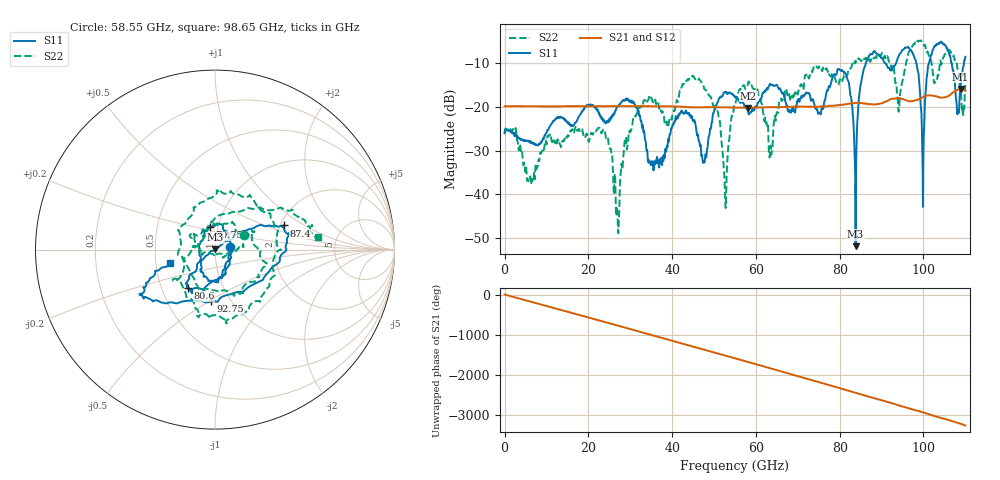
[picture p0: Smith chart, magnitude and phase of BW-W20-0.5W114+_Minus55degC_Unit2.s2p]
!Mini-Circuits Laboratory
!S-Parameters
!Model: BW-W20-0.5W114+
!Run / Lot / Date Code: QN2409253 /  / N/A
!Fixture:
!Network Analyzer: PNA-X N5242B - 423 4 ports (COM/DCOM);  Serial number: 74408
!Date: 3/8/2024 at 1:33:00 PM
!No.: Unit# 4 (U2  -55C)
!Tested with:
# Hz  S  dB  R  50
!Frequency  S11 dB  S11 Deg  S21 dB  S21 Deg  S12 dB  S12 Deg  S22 dB  S22 Deg
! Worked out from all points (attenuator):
!   2208 points, 10 MHz to 110 GHz, reference 50 ohm
!   highest |S21| = -15.86 dB at 108.8 GHz (marker M1); lowest = -20.2 dB at 58.2 GHz (marker M2)
!   lowest |S11| = -51.9 dB at 83.8 GHz (marker M3), VSWR 1.01, Z = 50.2 + j0.0672 ohm
!   |S11| at or under -10 dB: start of sweep to 86.23 GHz; 98.3 GHz to 101.3 GHz (3.014 GHz wide, 3.02 % of centre); 106.8 GHz to 109.6 GHz (2.884 GHz wide, 2.67 % of centre)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
!   |S22| runs from -48.9 to -4.7 dB; largest |S21 - S12| = 0.054
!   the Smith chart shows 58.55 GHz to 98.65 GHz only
!   S11 on the Smith chart (normalised r, x): 58.55 GHz: 1.18, +0.03; 70.75 GHz: 0.92, +0.23; 80.6 GHz: 0.68, -0.31; 87.4 GHz: 2.10, +0.68; 92.75 GHz: 0.82, -0.51; 98.65 GHz: 0.60, -0.09
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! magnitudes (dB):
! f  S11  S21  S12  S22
! 10 MHz  -26.0  -19.8  -19.8  -25.9
! 18.35 GHz  -21.3  -19.8  -19.8  -25.1
! 27 GHz  -19.9  -19.8  -19.8  -46.1
! 36.7 GHz  -32.3  -19.8  -19.8  -18.9
! 46.8 GHz  -28.6  -20.1  -20.1  -14.0
! 52.7 GHz  -16.6  -20.1  -20.1  -42.4
! 55.05 GHz  -17.6  -20.1  -20.1  -19.3
! 58.2 GHz  -21.4  -20.2  -20.2  -14.3
! 58.55 GHz  -21.4  -20.2  -20.2  -14.7
! 63.5 GHz  -15.0  -20.0  -20.0  -28.8
! 70.75 GHz  -17.9  -19.9  -19.9  -14.8
! 73.35 GHz  -18.2  -19.9  -19.9  -12.0
! 80.6 GHz  -11.6  -19.5  -19.6  -14.1
! 83.8 GHz  -51.9  -19.0  -19.2  -9.4
! 87.4 GHz  -7.8  -19.3  -19.2  -9.4
! 91.7 GHz  -11.0  -18.4  -18.5  -9.3
! 92.75 GHz  -10.8  -18.1  -18.3  -11.0
! 98.65 GHz  -11.7  -18.3  -18.4  -4.8
! 99.8 GHz  -34.1  -17.7  -17.9  -5.4
! 102.8 GHz  -5.9  -17.5  -17.6  -14.3
! 108.8 GHz  -15.7  -15.9  -15.8  -16.8
! 110 GHz  -8.5  -16.3  -16.2  -14.9
